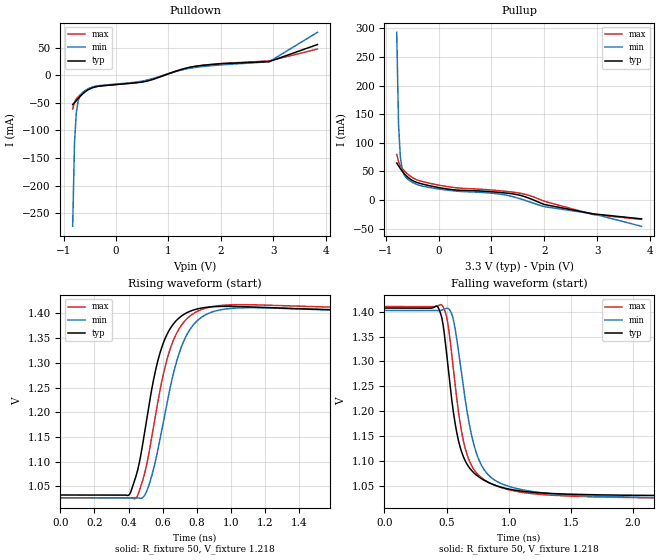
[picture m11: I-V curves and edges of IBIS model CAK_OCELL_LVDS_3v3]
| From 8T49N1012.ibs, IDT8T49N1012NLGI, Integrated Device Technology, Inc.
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[Model] CAK_OCELL_LVDS_3v3
Model_type   Output
Polarity   Non-Inverting
|   typ   min   max
C_comp   2pF   1.5pF   2.5pF
Vmeas = 1.241V
Rref = 50
Cref = 0
Vref = 1.241V
|   typ   min   max
[Voltage range]   3.3V   3.135V   3.465V
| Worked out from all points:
|   slope of the pulldown table from 0 to 0.495 V, typ, clamps not added: 108 ohm
|   slope of the pullup table from 0 to 0.495 V, typ, clamps not added: 98.2 ohm
|   rising waveform, R_fixture 50, V_fixture 1.218: 20-80 % time 126ps typ, 144ps min, 136ps max; typ from 1.03 V to 1.41 V
|   falling waveform, R_fixture 50, V_fixture 1.218: 20-80 % time 146ps typ, 172ps min, 147ps max; typ from 1.41 V to 1.03 V
[Pulldown]
|Voltage   I (typ)   I (min)   I (max)
|Note, modeling breaks down at 250mA and above.  This is well beyond the functional   |
|operating range of the device.  Should this scenario occur, catastrophic failure and   |
|possible damage to the device and/or board is of higher concern than the I-V curve   |
|behavior.  The IBIS checker will flag currents in excess of 10A with warnings.  Lines   |
|with currents in excess of 0.35 A have been commented out.  The points still remain|
|available to the user if the user desires to use them.   |
|-2.84000e+00   -2.67228e+01   -1.89425e+01   -2.18359e+01
|-2.38000e+00   -2.01823e+01   -1.46714e+01   -1.67120e+01
|-1.92000e+00   -1.36378e+01   -1.03985e+01   -1.15849e+01
|-1.46000e+00   -7.09099e+00   -6.12573e+00   -6.45782e+00
|-1.00000e+00   -5.49062e-01   -1.85643e+00   -1.33191e+00
|-9.99000e-01   -5.34865e-01   -1.84716e+00   -1.32078e+00
|-9.64529e-01   -1.74485e-01   -1.52731e+00   -9.37176e-01
|-9.30057e-01   -8.44549e-02   -1.20752e+00   -5.53760e-01
|-8.95586e-01   -6.39495e-02   -8.87799e-01   -2.24730e-01
|-8.61115e-01   -5.72064e-02   -5.68176e-01   -9.88520e-02
-826.6mV  -53.17mA   -273.7mA   -61.33mA
-792.2mV  -49.58mA   -122.3mA   -48.68mA
-757.7mV  -45.94mA   -67.64mA   -42.95mA
-723.2mV  -42.28mA   -46.73mA   -39.15mA
-688.8mV  -38.76mA   -37.71mA   -35.99mA
-619.8mV  -32.44mA   -29.86mA   -30.55mA
-516.4mV  -25.5mA    -23.75mA   -24.35mA
-378.5mV  -20.78mA   -19.56mA   -20.24mA
552.2mV   -11.35mA   -9.567mA   -10.56mA
1.483V    15.82mA    13.8mA     15.69mA
2.921V    24.74mA    24.53mA    26.06mA
3.841V    55.68mA    77.87mA    47.46mA
| 4.76040e+00   1.23653e+01   1.33136e+01   8.12971e+00
| 5.68020e+00   3.48096e+01   2.79570e+01   2.56901e+01
| 6.60000e+00   5.72931e+01   4.26336e+01   4.32888e+01
[Pullup]
|Voltage   I (typ)   I (min)   I (max)
|Note, modeling breaks down at 250mA and above.  This is well beyond the functional   |
|operating range of the device.  Should this scenario occur, catastrophic failure and   |
|possible damage to the device and/or board is of higher concern than the I-V curve   |
|behavior.  The IBIS checker will flag currents in excess of 10A with warnings.  Lines   |
|with currents in excess of 0.35 A have been commented out.  The points still remain|
|available to the user if the user desires to use them.   |
|-2.84000e+00   4.60704e+01   3.26954e+01   4.21827e+01
|-2.38000e+00   3.48230e+01   2.53572e+01   3.23205e+01
|-1.92000e+00   2.35813e+01   1.80254e+01   2.24641e+01
|-1.46000e+00   1.23556e+01   1.07001e+01   1.26178e+01
|-1.00000e+00   1.14497e+00   3.38771e+00   2.79054e+00
|-9.99000e-01   1.12061e+00   3.37184e+00   2.76919e+00
|-9.64529e-01   4.09746e-01   2.82468e+00   2.03340e+00
|-9.30057e-01   1.43694e-01   2.27764e+00   1.29778e+00
|-8.95586e-01   8.93474e-02   1.73071e+00   6.20278e-01
|-8.61115e-01   7.56244e-02   1.18387e+00   2.34858e-01
|-8.26644e-01   6.95173e-02   6.60281e-01   1.14826e-01
-792.2mV  64.66mA    293mA      79.43mA
-757.7mV  59.74mA    131.8mA    66.69mA
-723.2mV  54.85mA    75.02mA    60.06mA
-688.8mV  50.41mA    53.65mA    55.37mA
-585.3mV  40.06mA    36.35mA    45.25mA
-378.5mV  29.64mA    26.03mA    34.12mA
-33.8mV   22.29mA    19.71mA    26.61mA
1.276V    12.1mA     8.486mA    15.01mA
1.586V    7.045mA    758.4uA    11mA
2.001V    -7.892mA   -11.68mA   -2.205mA
2.921V    -24.19mA   -24.13mA   -25.41mA
3.841V    -33mA      -46.02mA   -33.99mA
|4.76040e+00   -7.07106e+00   -7.62874e+00   -5.15696e+00
|5.68020e+00   -2.01413e+01   -1.61596e+01   -1.66170e+01
|6.60000e+00   -3.32166e+01   -2.46965e+01   -2.80864e+01
[Ramp]
|   typ   min   max
dV/dt_r   0.229/0.132n   0.231/0.153n   0.235/0.143n
dV/dt_f   0.228/0.146n   0.229/0.172n   0.233/0.147n
R_load =   50.0000
[Rising Waveform]
R_fixture = 50
V_fixture   =1.218  |Vcc_typ
V_fixture_min=1.211  |Vcc_min
V_fixture_max=1.216  |Vcc_max
C_fixture = 0.0p
| Time   typ   min   max
0s        1.033V     1.027V     1.027V
400ps     1.032V     1.027V     1.027V
448.9ps   1.077V     1.027V     1.029V
488.9ps   1.147V     1.029V     1.069V
568.9ps   1.3V       1.118V     1.214V
653.3ps   1.374V     1.263V     1.336V
742.2ps   1.401V     1.356V     1.389V
857.8ps   1.412V     1.398V     1.411V
1.111ns   1.413V     1.411V     1.417V
4ns       1.405V     1.399V     1.408V
[Falling Waveform]
R_fixture = 50
V_fixture   =1.218  |Vcc_typ
V_fixture_min=1.211  |Vcc_min
V_fixture_max=1.216  |Vcc_max
C_fixture = 0.0p
| Time   typ   min   max
0s        1.407V     1.402V     1.41V
426.7ps   1.41V      1.402V     1.411V
471.1ps   1.375V     1.404V     1.41V
528.9ps   1.25V      1.402V     1.342V
591.1ps   1.146V     1.33V      1.208V
666.7ps   1.093V     1.197V     1.111V
764.4ps   1.067V     1.1V       1.07V
906.7ps   1.05V      1.059V     1.049V
1.604ns   1.032V     1.03V      1.028V
4ns       1.031V     1.024V     1.025V
